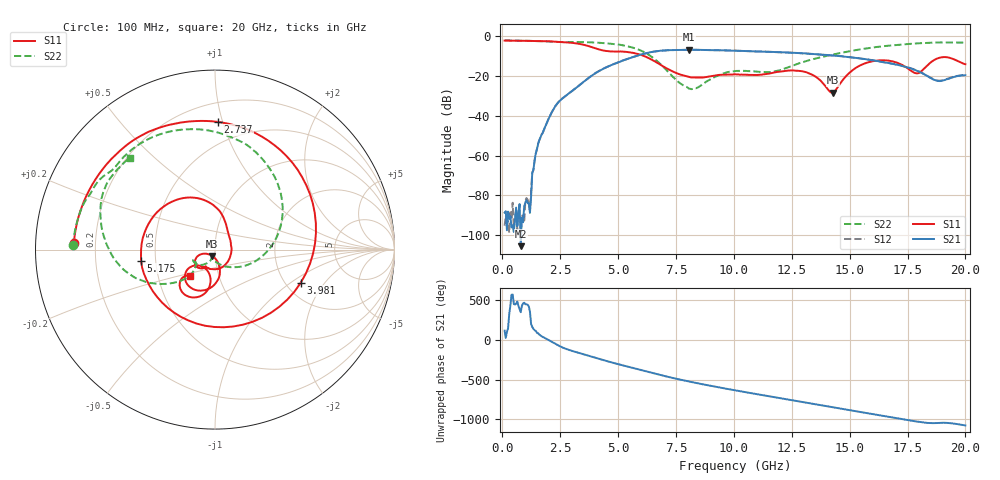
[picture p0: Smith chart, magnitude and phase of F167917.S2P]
!  2-Port S-parameters saved by WinCal
! VAR MeasName=S-Parameters (CALIBRATED_DATA) read from VNA (N5242A)
! VAR MeasDate=2016-11-22 8:59:24
! VAR NAME=F167917
! VAR FILENAME=F167917.S2P
! VAR DATE=2016-11-22 8:59:24
! VAR PHYS_PORTS=1,2
# Hz S DB R 50
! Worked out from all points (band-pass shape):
!   401 points, 100 MHz to 20 GHz, reference 50 ohm
!   highest |S21| = -6.68 dB at 8.06 GHz (marker M1); lowest = -105.5 dB at 796.5 MHz (marker M2)
!   |S21| within 3 dB of the highest: 5.833 GHz to 14.35 GHz (8.514 GHz wide, 84.4 % of centre)
!   lowest |S11| = -28.3 dB at 14.28 GHz (marker M3), VSWR 1.08, Z = 48.3 - j3.37 ohm
!   |S11| at or under -10 dB: 6.151 GHz to end of sweep
!   |S22| runs from -26.5 to -2.0 dB; largest |S21 - S12| = 0.0053
!   S11 on the Smith chart (normalised r, x): 100 MHz: 0.12, +0.02; 2.737 GHz: 0.34, +0.97; 3.981 GHz: 2.39, -1.21; 5.175 GHz: 0.41, -0.06; 20 GHz: 0.73, -0.22
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1e8  -2.09 177.3  -88.67 117.2  -95.25 82.6  -2.03 178.3
7.965e8  -2.19 158.8  -105.54 -9.9  -89.45 178.1  -2.13 167.2
1.14475e9  -2.25 149.1  -83.94 65.1  -83.85 67.1  -2.20 161.5
1.64225e9  -2.34 134.0  -50.98 58.0  -50.93 56.7  -2.39 153.9
2.23925e9  -2.58 111.7  -36.04 -40.2  -36.01 -40.8  -2.73 144.0
2.73675e9  -2.95 88.6  -29.90 -111.5  -29.90 -111.9  -2.81 137.2
3.43325e9  -4.00 39.6  -23.59 -174.3  -23.60 -174.4  -2.84 123.5
3.9805e9  -5.82 -21.3  -18.80 138.5  -18.78 138.7  -3.06 110.2
4.478e9  -7.31 -90.5  -15.64 95.7  -15.58 95.6  -3.45 96.2
5.1745e9  -7.60 -171.5  -12.26 41.6  -12.22 41.2  -4.39 71.3
5.92075e9  -9.04 128.9  -9.36 -14.3  -9.37 -14.8  -6.80 34.9
6.7665e9  -13.78 80.2  -7.27 -78.5  -7.31 -78.7  -13.24 -20.2
8.06e9  -20.31 24.1  -6.68 -164.9  -6.69 -164.9  -26.29 -111.2
1.005e10  -19.03 -104.5  -7.16 83.5  -7.16 83.6  -17.48 -146.2
1.1642e10  -18.41 -121.9  -7.79 2.4  -7.77 2.4  -17.80 -146.9
1.338325e10  -19.27 -157.9  -8.79 -85.6  -8.79 -85.4  -11.54 -138.3
1.427875e10  -28.32 -115.0  -9.57 -130.6  -9.59 -130.2  -9.11 -146.9
1.537325e10  -15.09 -86.2  -10.96 174.1  -10.92 174.4  -6.66 -159.7
1.67165e10  -12.25 -130.6  -13.44 107.5  -13.41 107.8  -4.61 -179.4
1.79105e10  -18.61 -122.0  -17.32 48.6  -17.17 48.6  -3.52 163.0
1.895525e10  -10.53 -116.9  -22.39 33.1  -22.19 32.8  -3.02 146.5
2e10  -13.98 -133.2  -19.49 -0.5  -19.33 -0.6  -3.11 132.8
